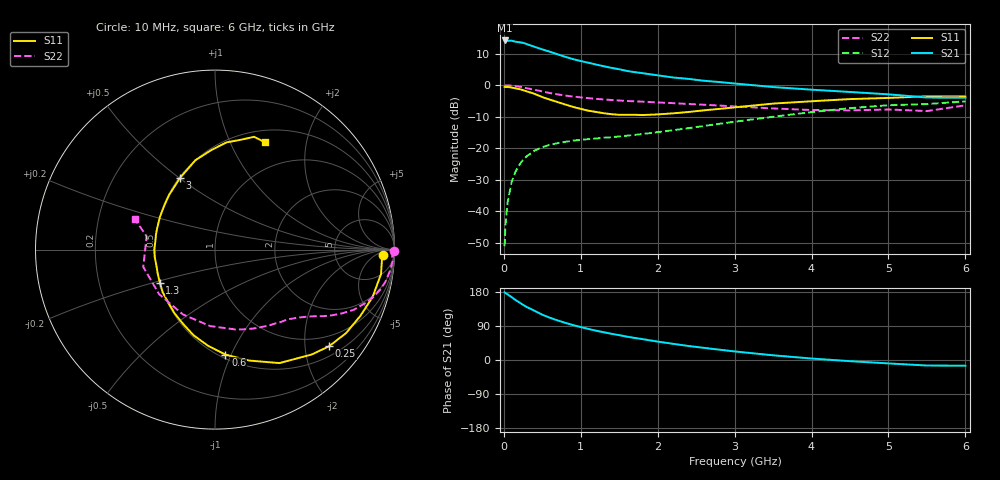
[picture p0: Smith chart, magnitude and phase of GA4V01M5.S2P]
! Infineon Technologies  Discrete & RF Semiconductors
! BF775
! Si NPN RF Bipolar Junction Transistor in SOT23
! VCE = 4 V  IC = 1.5 mA
! Common Emitter S-Parameters:  May  1996
# GHz  S  MA  R  50
!  f  S11  S21  S12  S22
! GHz  MAG  ANG  MAG  ANG  MAG  ANG  MAG  ANG
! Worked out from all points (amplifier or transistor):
!   36 points, 10 MHz to 6 GHz, reference 50 ohm
!   highest |S21| = 14.2 dB at 10 MHz (marker M1)
!   |S21| within 3 dB of that: start of sweep to 520.9 MHz
!   unconditionally stable (mu >= 1): 1.297 GHz to 3.752 GHz; 5.257 GHz to end of sweep
!   at 250 MHz: K = 0.24, MSG = 18.5 dB, |S12| = -23.7 dB
!   at 1.4 GHz: K = 1.06, MAG = 9.5 dB, |S12| = -16.5 dB
!   at 6 GHz: K = 1.00, MAG = 0.5 dB, |S12| = -5.2 dB
!   S11 on the Smith chart (normalised r, x): 10 MHz: 25, -12; 250 MHz: 0.72, -2.55; 600 MHz: 0.53, -0.95; 1.3 GHz: 0.50, -0.21; 3 GHz: 0.51, +0.50; 6 GHz: 0.64, +1.36
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0.01  0.9381 -1.8  5.106 178.8  0.0028 88.1  0.9995 -0.6
0.02  0.9319 -3.5  5.067 177.0  0.0058 88.2  0.9862 -1.4
0.05  0.935 -8.4  5.046 173.0  0.0142 84.5  0.9924 -3.6
0.1  0.9167 -16.8  5.064 166.1  0.0287 80.4  0.9811 -7.1
0.15  0.8902 -24.5  4.883 158.6  0.042 74.9  0.9664 -10.7
0.25  0.8329 -40.3  4.68 145.5  0.0655 66.5  0.921 -16.6
0.3  0.7951 -47.3  4.464 139.6  0.075 63.2  0.8923 -19.3
0.4  0.7272 -60.4  4.044 129.7  0.0916 56.7  0.8432 -23.4
0.5  0.6472 -72.8  3.679 119.5  0.1042 51.8  0.7929 -26.6
0.6  0.588 -84.3  3.381 111.4  0.1132 48.1  0.7482 -29.3
0.8  0.4919 -104.1  2.806 98.0  0.1263 43.1  0.6819 -32.9
0.9  0.4519 -112.9  2.582 92.1  0.132 41.8  0.6595 -34.3
1.1  0.3927 -131.9  2.263 82.0  0.1393 40.4  0.6215 -37.2
1.3  0.3582 -149.0  1.991 73.2  0.1466 40.4  0.5922 -39.8
1.7  0.3386 179.7  1.607 58.2  0.1626 42.1  0.5531 -45.7
2.2  0.3569 149.4  1.321 42.7  0.1927 44.9  0.5183 -54.8
3  0.4438 116.2  1.061 22.6  0.2629 45.2  0.4599 -75.5
3.5  0.5097 102.4  0.932 12.4  0.3152 41.8  0.427 -93.6
4.5  0.6006 83.9  0.779 -3.1  0.4312 30.2  0.3983 -141.4
5  0.627 77.1  0.714 -9.0  0.4803 22.4  0.4112 -166.4
5.5  0.6649 70.9  0.636 -14.6  0.5013 13.6  0.3879 169.0
6  0.6599 65.1  0.631 -15.0  0.5523 8.9  0.4784 159.2
